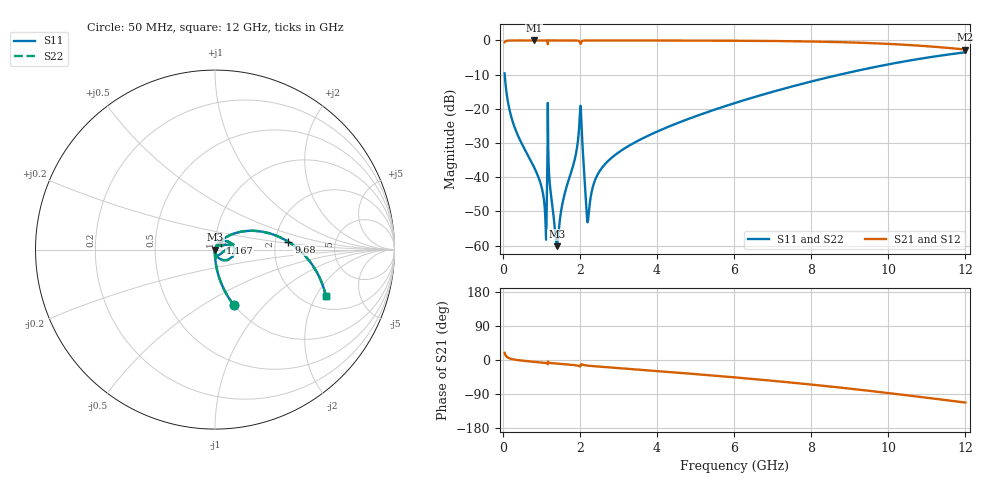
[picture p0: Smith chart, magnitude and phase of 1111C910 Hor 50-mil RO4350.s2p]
# GHz S MA R 50
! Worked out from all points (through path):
!   11951 points, 50 MHz to 12 GHz, reference 50 ohm
!   highest |S21| = -0.01 dB at 811 MHz (marker M1); lowest = -2.7 dB at 12 GHz (marker M2)
!   group delay of S21, straight-line fit = 26 ps
!   lowest |S11| = -60.2 dB at 1.403 GHz (marker M3), VSWR 1.00, Z = 50.1 - j0.017 ohm
!   |S11| at or under -10 dB: 52.23 MHz to 8.743 GHz (8.691 GHz wide, 198 % of centre)
!   |S22| runs from -60.2 to -3.5 dB; largest |S21 - S12| = 0
!   S11 on the Smith chart (normalised r, x): 50 MHz: 1.00, -0.70; 1.167 GHz: 1.06, +0.08; 9.68 GHz: 2.37, +0.25; 12 GHz: 2.58, -2.43
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0.05  0.3289 -71.1  0.9441 18.9  0.9441 18.9  0.3289 -71.1
0.282  0.05932 -88.0  0.9977 1.5  0.9977 1.5  0.05932 -88.0
0.811  0.0141 -91.6  0.9991 -4.7  0.9991 -4.7  0.0141 -91.6
0.998  0.007537 -89.7  0.999 -6.3  0.999 -6.3  0.007537 -89.7
1.088  0.003722 -81.8  0.9989 -7.1  0.9989 -7.1  0.003722 -81.8
1.167  0.05003 51.8  0.9756 -10.4  0.9756 -10.4  0.05003 51.8
1.215  0.008862 -91.2  0.9989 -7.7  0.9989 -7.7  0.008862 -91.2
1.403  0.0009782 -10.0  0.9989 -9.5  0.9989 -9.5  0.0009782 -10.0
1.585  0.005076 66.4  0.9988 -11.0  0.9988 -11.0  0.005076 66.4
1.885  0.01994 68.7  0.9971 -13.8  0.9971 -13.8  0.01994 68.7
1.988  0.05943 50.0  0.9747 -16.5  0.9747 -16.5  0.05943 50.0
2.042  0.06375 -59.3  0.9564 -11.0  0.9564 -11.0  0.06375 -59.3
2.158  0.004683 -66.8  0.997 -14.3  0.997 -14.3  0.004683 -66.8
2.216  0.002396 17.0  0.9978 -14.9  0.9978 -14.9  0.002396 17.0
2.381  0.008596 63.6  0.9983 -16.4  0.9983 -16.4  0.008596 63.6
2.638  0.01514 66.3  0.9984 -18.5  0.9984 -18.5  0.01514 66.3
4.034  0.04718 58.6  0.997 -29.4  0.997 -29.4  0.04718 58.6
6.025  0.1215 43.0  0.99 -45.9  0.99 -45.9  0.1215 43.0
8.017  0.2519 24.3  0.9641 -64.9  0.9641 -64.9  0.2519 24.3
9.68  0.4112 6.0  0.9069 -83.4  0.9069 -83.4  0.4112 6.0
10.009  0.4472 2.1  0.8896 -87.3  0.8896 -87.3  0.4472 2.1
12  0.6703 -22.8  0.7359 -112.3  0.7359 -112.3  0.6703 -22.8
